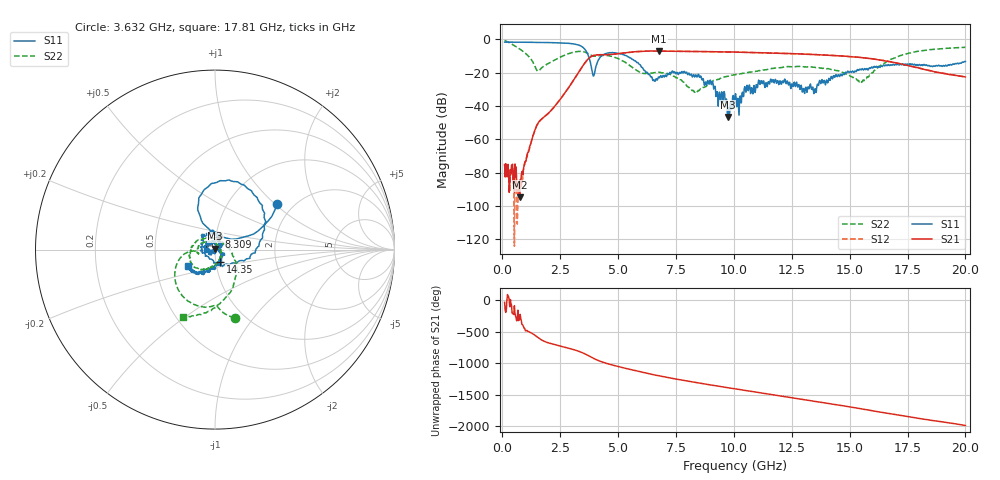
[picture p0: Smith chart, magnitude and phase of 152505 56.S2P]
!  2-Port S-parameters saved by WinCal
! VAR MeasName=S-Parameters (CALIBRATED_DATA) read from VNA (N5230C)
! VAR MeasDate=4/10/2015 9:34:21 AM
! VAR NAME=152505 56
! VAR FILENAME=152505 56.S2P
! VAR DATE=4/10/2015 9:34:21 AM
! VAR PHYS_PORTS=1,2
# Hz S DB R 50
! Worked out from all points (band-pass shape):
!   801 points, 100 MHz to 20 GHz, reference 50 ohm
!   highest |S21| = -7.09 dB at 6.766 GHz (marker M1); lowest = -94.7 dB at 746.8 MHz (marker M2)
!   |S21| within 3 dB of the highest: 3.879 GHz to 14.67 GHz (10.79 GHz wide, 116 % of centre)
!   lowest |S11| = -46.6 dB at 9.727 GHz (marker M3), VSWR 1.01, Z = 50.1 + j0.462 ohm
!   |S11| at or under -10 dB: 3.72 GHz to 4.296 GHz (576 MHz wide, 14.4 % of centre); 5.37 GHz to end of sweep
!   |S22| runs from -31.8 to -0.8 dB; largest |S21 - S12| = 0.0055
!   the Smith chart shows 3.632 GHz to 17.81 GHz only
!   S11 on the Smith chart (normalised r, x): 3.632 GHz: 1.66, +1.03; 8.309 GHz: 1.03, +0.15; 14.35 GHz: 1.05, -0.14; 17.81 GHz: 0.73, -0.14
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1e8  -1.75 177.6  -75.08 -33.6  -75.01 -17.0  -0.75 -18.8
7.4675e8  -1.80 162.2  -94.70 48.3  -93.53 54.9  -5.84 -103.5
1.54275e9  -1.92 142.0  -50.43 126.7  -50.49 126.1  -19.17 171.1
2.23925e9  -2.09 121.3  -40.60 17.0  -40.70 16.2  -12.69 74.5
3.43325e9  -4.41 57.4  -16.88 -108.9  -16.93 -108.7  -7.34 -54.7
3.63225e9  -7.38 36.1  -13.03 -142.6  -13.06 -142.6  -8.09 -73.9
3.93075e9  -22.02 66.4  -9.80 159.2  -9.82 159.3  -10.04 -88.1
4.42825e9  -8.79 94.2  -9.27 86.2  -9.30 86.0  -9.69 -110.6
5.398375e9  -10.32 26.0  -8.03 -7.6  -8.03 -7.6  -14.67 -169.6
6.741625e9  -22.66 -166.2  -7.10 -118.2  -7.09 -118.4  -19.76 -174.6
6.7665e9  -22.69 -165.1  -7.09 -119.9  -7.10 -120.1  -19.83 -175.1
8.30875e9  -22.67 73.5  -7.38 137.5  -7.40 137.6  -31.84 50.9
9.079875e9  -25.30 47.2  -7.54 90.5  -7.50 90.7  -25.16 -56.9
9.726625e9  -46.59 80.4  -7.65 52.3  -7.62 52.3  -22.24 -85.1
1.005e10  -34.29 -119.8  -7.71 33.2  -7.74 33.2  -21.34 -90.4
1.116938e10  -24.99 -177.0  -8.14 -30.9  -8.10 -30.9  -18.62 -111.2
1.338325e10  -29.22 20.2  -9.15 -157.0  -9.11 -156.8  -16.61 -167.0
1.435338e10  -22.85 -67.4  -9.80 145.9  -9.79 146.1  -18.54 161.8
1.55225e10  -17.93 -107.9  -11.04 74.7  -11.01 74.5  -25.82 56.1
1.669162e10  -15.32 -127.0  -13.36 1.1  -13.36 0.3  -12.67 -64.4
1.7811e10  -15.01 -148.9  -16.75 -65.8  -16.76 -67.0  -7.66 -115.6
2e10  -13.37 -146.0  -22.65 172.3  -22.64 172.8  -4.83 -176.5
